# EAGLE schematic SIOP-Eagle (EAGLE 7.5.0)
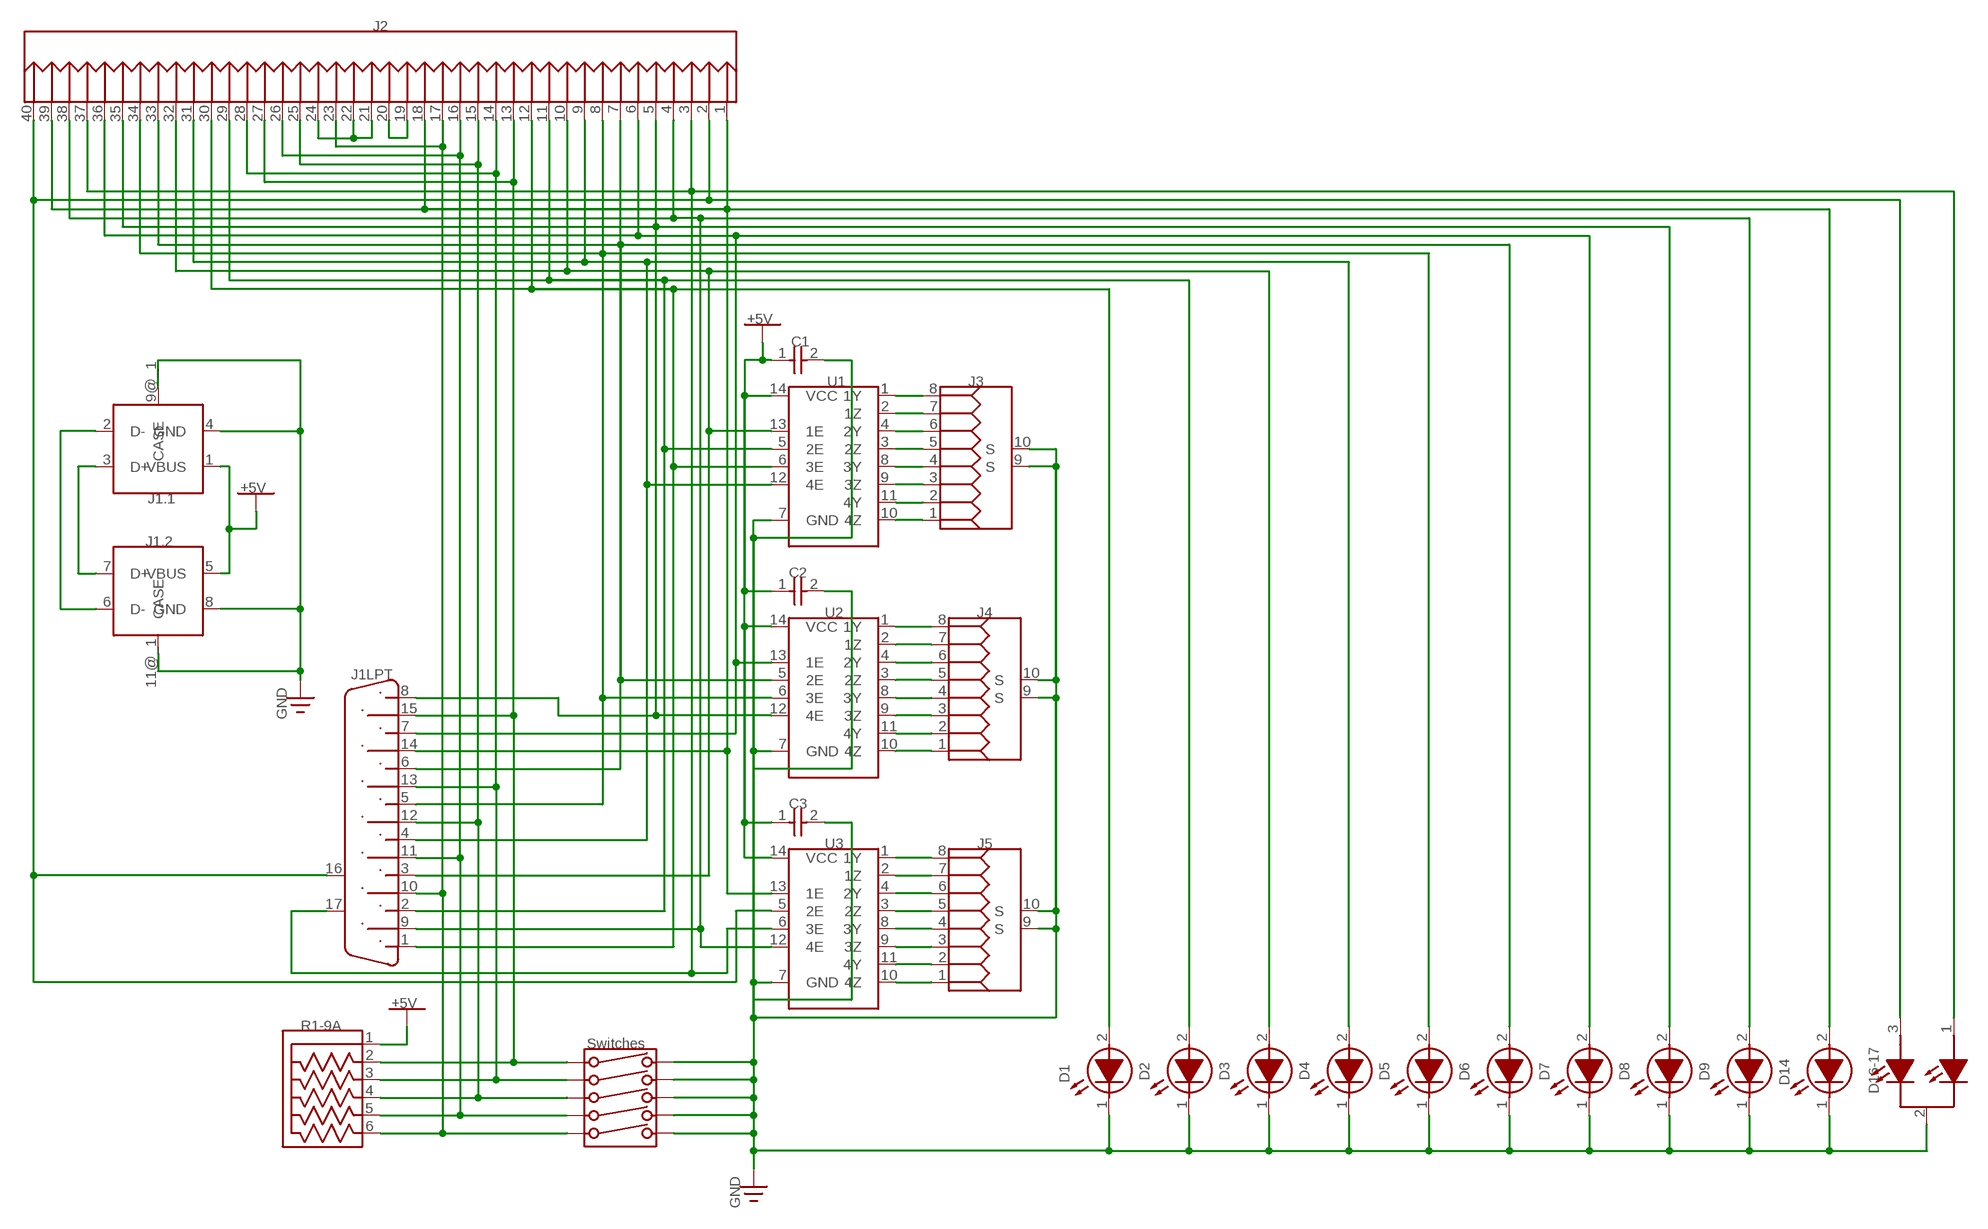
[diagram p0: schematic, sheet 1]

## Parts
C1  0.1uF  0402B104K160NT  [CAPC100X50X55L25N_AD3]
C2  0.1uF  0402B104K160NT  [CAPC100X50X55L25N_AD3]
C3  0.1uF  0402B104K160NT  [CAPC100X50X55L25N_AD3]
D1  LED-2X5MM_RECTANGULAR_RED  [LED-2X5MM_RECTANGULAR_RED]
D2  LED-2X5MM_RECTANGULAR_RED  [LED-2X5MM_RECTANGULAR_RED]
D3  LED-2X5MM_RECTANGULAR_RED  [LED-2X5MM_RECTANGULAR_RED]
D4  LED-2X5MM_RECTANGULAR_RED  [LED-2X5MM_RECTANGULAR_RED]
D5  LED-2X5MM_RECTANGULAR_RED  [LED-2X5MM_RECTANGULAR_RED]
D6  LED-2X5MM_RECTANGULAR_RED  [LED-2X5MM_RECTANGULAR_RED]
D7  LED-2X5MM_RECTANGULAR_RED  [LED-2X5MM_RECTANGULAR_RED]
D8  LED-2X5MM_RECTANGULAR_RED  [LED-2X5MM_RECTANGULAR_RED]
D9  LED-2X5MM_RECTANGULAR_RED  [LED-2X5MM_RECTANGULAR_RED]
D14  LED-2X5MM_RECTANGULAR_RED  [LED-2X5MM_RECTANGULAR_RED]
D16-17  LED-8MM_ROUND_BI-COLOR  [LED-8MM_ROUND_BI-COLOR]
J1  Type A, Receptacle  292323-1  [TE_292323-1]
J1LPT  788757-2  [DSUB-1.385/2H15]
J2  SBH31-NBPB-D20-ST-BK  [SHDRV40W45P127_20X2_2840X535H560]
J3  R-RJ45R10P-B000  [CKMTW_RJ45-TH_R-RJ45R10P-B000]
J4  R-RJ45R10P-B000  [CKMTW_RJ45-TH_R-RJ45R10P-B000]
J5  R-RJ45R10P-B000  [CKMTW_RJ45-TH_R-RJ45R10P-B000]
R1-9A  RES6SIPB  [SIP-6/16.5X2.4X2.54]
Switches  SWITCH_5DIP  (no package)
U1  CD74HC4066E  [DIP794W45P254L1969H508Q14]
U2  CD74HC4066E  [DIP794W45P254L1969H508Q14]
U3  CD74HC4066E  [DIP794W45P254L1969H508Q14]

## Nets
Net_0: J3.8 U1.1(1Y)
Net_1: J3.7 U1.2(1Z)
Net_2: J3.6 U1.4(2Y)
Net_3: J3.5 U1.3(2Z)
Net_4: J3.4 U1.8(3Y)
Net_5: J3.3 U1.9(3Z)
Net_6: J3.2 U1.11(4Y)
Net_7: J3.1 U1.10(4Z)
Net_8: J4.8 U2.1(1Y)
Net_9: J4.7 U2.2(1Z)
Net_10: J4.6 U2.4(2Y)
Net_11: J4.5 U2.3(2Z)
Net_12: J4.4 U2.8(3Y)
Net_13: J4.3 U2.9(3Z)
Net_14: J4.2 U2.11(4Y)
Net_15: J4.1 U2.10(4Z)
Net_16: J5.8 U3.1(1Y)
Net_17: J5.7 U3.2(1Z)
Net_18: J5.6 U3.4(2Y)
Net_19: J5.5 U3.3(2Z)
Net_20: J5.4 U3.8(3Y)
Net_21: J5.3 U3.9(3Z)
Net_22: J5.2 U3.11(4Y)
Net_23: J5.1 U3.10(4Z)
Net_24: C1.1 C2.1 C3.1 J1.1(PART_1:VBUS) J1.5(PART_2:VBUS) R1-9A.1 U1.14(VCC) U2.14(VCC) U3.14(VCC) ; supply symbol labelled +5V
Net_25: C1.2 C2.2 C3.2 D1.1(K) D2.1(K) D3.1(K) D4.1(K) D5.1(K) D6.1(K) D7.1(K) D8.1(K) D9.1(K) D14.1(K) D16-17.2(K_Common) J1.4(PART_1:GND) J1.8(PART_2:GND) J1.9@_1(PART_1:CASE) J1.11@_1(PART_2:CASE) J3.9(S) J3.10(S) J4.9(S) J4.10(S) J5.9(S) J5.10(S) Switches.6 Switches.7 Switches.8 Switches.9 Switches.10 U1.7(GND) U2.7(GND) U3.7(GND) ; supply symbol labelled GND
Net_28: D4.2(A) J1LPT.4 J2.9 J2.31 U1.12(4E)
Net_29: D3.2(A) J1LPT.3 J2.10 J2.32 U1.13(1E)
Net_30: D1.2(A) J1LPT.1 J2.12 J2.30 U1.6(3E)
Net_31: D9.2(A) J1LPT.9 J2.4 J2.38 U3.12(4E)
Net_32: D7.2(A) J1LPT.7 J2.6 J2.36 U2.13(1E)
Net_33: J1LPT.15 J2.13 J2.27 R1-9A.2 Switches.1
Net_34: J1LPT.13 J2.14 J2.28 R1-9A.3 Switches.2
Net_35: J2.19 J2.20
Net_36: J2.21 J2.22 J2.24
Net_37: J1.3(PART_1:D+) J1.7(PART_2:D+)
Net_38: D6.2(A) J1LPT.6 J2.7 J2.33 U2.5(2E)
Net_39: J1.2(PART_1:D-) J1.6(PART_2:D-)
Net_40: D8.2(A) J1LPT.8 J2.5 J2.35 U2.12(4E)
Net_47: D2.2(A) J1LPT.2 J2.11 J2.29 U1.5(2E)
Net_48: D5.2(A) J1LPT.5 J2.8 J2.34 U2.6(3E)
Net_49: J1LPT.12 J2.15 J2.25 R1-9A.4 Switches.3
Net_50: J1LPT.11 J2.16 J2.26 R1-9A.5 Switches.4
Net_51: J1LPT.10 J2.17 J2.23 R1-9A.6 Switches.5
Net_53: D14.2(A) J1LPT.14 J2.1 J2.18 J2.39 U3.13(1E)
Net_54: D16-17.3(A) J1LPT.16(MH1) J2.2 J2.40 U3.5(2E)
Net_55: D16-17.1(A) J1LPT.17(MH2) J2.3 J2.37 U3.6(3E)

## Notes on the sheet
- J2
- +5V
- C1
- U1 | J3
- J1.1 | +5V
- J1.2
- C2
- U2 | J4
- J1LPT
- GND
- C3
- U3 | J5
- +5V
- R1-9A
- Switches | D16-17
- D2 | D3 | D4 | D5 | D6 | D7 | D8 | D9 | D14
- D1
- GND

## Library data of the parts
C1-C3 = common:0402B104K160NT; DATASHEET: http://datasheets.diptrace.com/fh/0603F104M500NT_and_series.pdf; MANUFACTURER: FH(Guangdong Fenghua Advanced Tech); PART_NUMBER_(LCSC): C41851; UNIQUE_NAME: FH_0402(1005)
D1-D9 D14 = common:LED-2X5MM_RECTANGULAR_RED; DATASHEET: http://datasheets.diptrace.com/sensors_led/WP103HDT.pdf; MANUFACTURER: Kingbright; UNIQUE_NAME: KINGBRIGHT_LED-2X5RECT_RED
D16-17 = common:LED-8MM_ROUND_BI-COLOR; DATASHEET: http://datasheets.diptrace.com/sensors_led/WP799EGW.pdf; MANUFACTURER: Kingbright; UNIQUE_NAME: KINGBRIGHT_LED(BI)-8R
J1 = common:292323-1; DATASHEET: http://datasheets.diptrace.com/con_usb/292323.pdf; MANUFACTURER: TE Connectivity; PART_NUMBER_(DIGI-KEY): 292323-1-ND; PART_NUMBER_(MOUSER): 571-292323-1; UNIQUE_NAME: TE_292323-1
J1LPT = common:788757-2; MANUFACTURER: TE Connectivity; UNIQUE_NAME: TE_DSUB-1.385/2H15
J2 = common:SBH31-NBPB-D20-ST-BK; DATASHEET: http://datasheets.diptrace.com/con_headers/SBH31-NBPB-D___-ST-___11098-B.pdf; MANUFACTURER: Sullins; PART_NUMBER_(DIGI-KEY): S9091-ND; UNIQUE_NAME: SULLINS_SBH31-NBPB-D20-ST-BK
J3-J5 = common:R-RJ45R10P-B000; DATASHEET: http://datasheets.diptrace.com/ckmtw/R-RJ45R10P-B000.pdf; MANUFACTURER: Ckmtw(Shenzhen Cankemeng); PART_NUMBER_(LCSC): C386758; UNIQUE_NAME: CKMTW_RJ45-TH_R-RJ45R10P-B000
R1-9A = common:RES6SIPB; UNIQUE_NAME: SIP-6/16.5x2.4x2.54
Switches = common:SWITCH_5DIP; DESCRIPTION_1: DIP Switch; DESCRIPTION_2: 5 Positions
U1-U3 = common:CD74HC4066E; DATASHEET: http://datasheets.diptrace.com/ti/CDx4HC4066.pdf; MANUFACTURER: Texas Instruments; PART_NUMBER_(DIGI-KEY): 296-14533-5-ND; PART_NUMBER_(LCSC): C1546314; PART_NUMBER_(MOUSER): 595-CD74HC4066E; UNIQUE_NAME: TI_N_R-PDIP-T14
